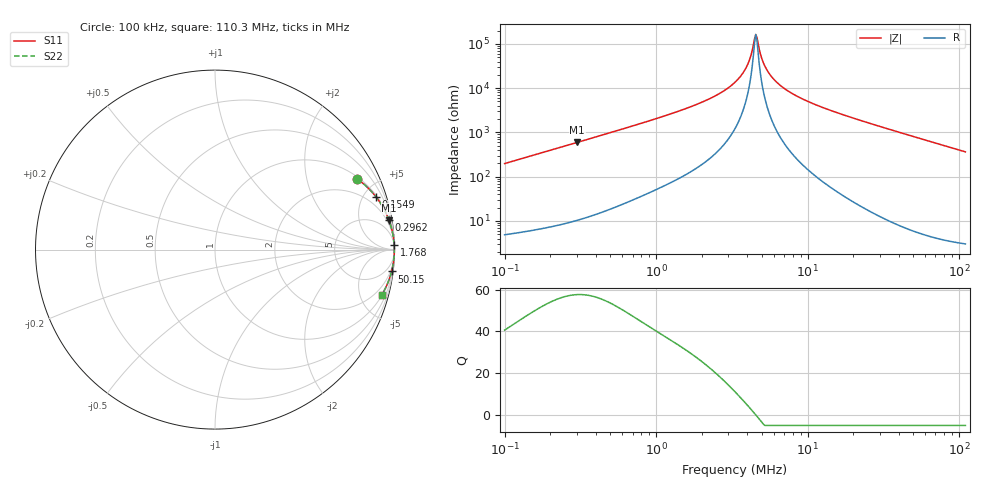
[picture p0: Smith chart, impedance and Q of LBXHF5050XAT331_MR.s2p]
! LBXHF5050XAT331_MR  S-PARAMETER MODEL  ( Standard Model )
! Model Generated by TAIYO YUDEN Corporation (http://www.ty-top.com)
! Version 1.0
! TAIYO YUDEN Control No. 20240926
! Copyright(c) 2024 TAIYO YUDEN CO.,LTD. All Rights Reserved.
! Product Description (link to TY-COMPAS)
! https://ds.yuden.co.jp/TYCOMPAS/or/detail?pn=LBXHF5050XAT331MMR&u=M
! Products Name : Inductors
! Characteristics :
!  Inductance : 330 [uH] , SRF(min) : 3.0 [MHz] , DC Resistance(max) : 2.76 [Ohm]
!  Rated Current : Saturation  300 [mA] , Temp Rise  190 [mA] (20 [degC])
!  Case Size : 5.0 x 5.0 / 0.197 x 0.197 [mm/inch] , Thickness : 3.1 / 0.122 [mm/inch]
!  (Conditions: Temperature = 25 [degC] , DC Bias Current = 0 [A])
! External Node Assignments :
!  1  o---GGG---o  2
! GND o---------o GND
! Frequency Range : 0.1MHz  -  110.285862MHz  [ 402 STEP ]
# MHz S RI R 50
! Freq[MHz].  S11 Real  S11 Imag  S21 Real  S21 Imag  S12 Real  S12 Imag  S22 Real  S22 Imag
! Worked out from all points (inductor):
!   401 points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, 100 kHz to 110.3 MHz, reference 50 ohm
!   read as one part in series: L = 314 uH near 103.6 kHz
!   highest Q = 57.6 at 301.4 kHz (marker M1), where L = 314 uH
!   self-resonance near 4.552 MHz
!   S11 on the Smith chart (normalised r, x): 100 kHz: 1.10, +3.96; 154.9 kHz: 1.12, +6.12; 296.2 kHz: 1, +12; 1.768 MHz: 4, +81; 50.15 MHz: 1, -16; 110.3 MHz: 1.06, -7.28
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0.1  0.7908 0.3946  0.2092 -0.3946  0.2092 -0.3946  0.7908 0.3946
0.154938  0.8987 0.2919  0.1013 -0.2919  0.1013 -0.2919  0.8987 0.2919
0.296204  0.9688 0.1653  0.0312 -0.1653  0.0312 -0.1653  0.9688 0.1653
0.301437  0.9698 0.1626  0.0302 -0.1626  0.0302 -0.1626  0.9698 0.1626
0.323312  0.9735 0.1521  0.0265 -0.1521  0.0265 -0.1521  0.9735 0.1521
1.045308  0.9967 0.0463  0.00334 -0.0463  0.00334 -0.0463  0.9967 0.0463
1.7678  0.9985 0.0247  0.00148 -0.0247  0.00148 -0.0247  0.9985 0.0247
2.598793  0.9991 0.0134  0.0009 -0.0134  0.0009 -0.0134  0.9991 0.0134
3.320932  0.9993 0.00732  0.000713 -0.00732  0.000713 -0.00732  0.9993 0.00732
3.956607  0.9994 0.00324  0.000639 -0.00324  0.000639 -0.00324  0.9994 0.00324
4.170055  0.9994 0.00204  0.000625 -0.00204  0.000625 -0.00204  0.9994 0.00204
4.472672  0.9994 0.000446  0.000612 -0.000446  0.000612 -0.000446  0.9994 0.000446
4.551697  0.9994 4.85e-05  0.00061 -4.85e-05  0.00061 -4.85e-05  0.9994 4.85e-05
4.71396  0.9994 -0.000747  0.000606 0.000747  0.000606 0.000747  0.9994 -0.000747
4.968266  0.9994 -0.00194  0.000604 0.00194  0.000604 0.00194  0.9994 -0.00194
5.23629  0.9994 -0.00314  0.000606 0.00314  0.000606 0.00314  0.9994 -0.00314
5.919265  0.9994 -0.00599  0.000622 0.00599  0.000622 0.00599  0.9994 -0.00599
7.432753  0.9993 -0.0115  0.000709 0.0115  0.000709 0.0115  0.9993 -0.0115
10.73698  0.9989 -0.0219  0.00105 0.0219  0.00105 0.0219  0.9989 -0.0219
34.71395  0.9921 -0.0844  0.00789 0.0844  0.00789 0.0844  0.9921 -0.0844
50.14601  0.984 -0.122  0.016 0.122  0.016 0.122  0.984 -0.122
110.2859  0.928 -0.2543  0.072 0.2543  0.072 0.2543  0.928 -0.2543
